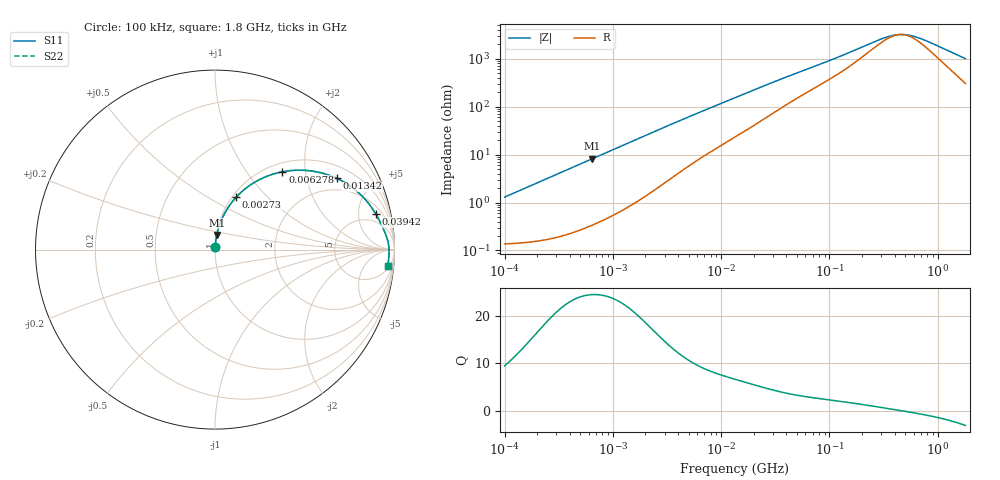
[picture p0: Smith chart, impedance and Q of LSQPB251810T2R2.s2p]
! LSQPB251810T2R2  S-PARAMETER MODEL  ( General Type )
! Model Generated by TAIYO YUDEN Corporation (http://www.ty-top.com)
! Version 2.0
! TAIYO YUDEN Control No. 100810NG22EB-FKC
! Copyright(c) 2009 TAIYO YUDEN CO.,LTD. All Rights Reserved.
! Product Description (link to TY-COMPAS)
! https://ds.yuden.co.jp/TYCOMPAS/or/detail?pn=LSQPB251810T2R2M&u=M
! Products Name : Inductors
! Characteristics :
!  Inductance : 2.2 uH , SRF(min) : 80 MHz , DC Resistance(max) : 0.169 Ohm
!  Rated Current : Saturation :850 mA , Temp Rise : 950 mA (40 degC)
!  Case Size : 2.5 x 1.8 / 0.098 x 0.071 [mm/inch] , Thickness : 1.0 / 0.04 [mm/inch]
!  (Conditions: Temperature = 25 degC , DC Bias Current/Voltage = 0A / 0V)
! External Node Assignments :
!  1  o---GGG---o  2
! GND o---------o GND
! Frequency Range : 0.1MHz  -  1800MHz  [ 402 STEP ]
# MHz S RI R 50
! Freq[MHz].  S11 Real  S11 Imag  S21 Real  S21 Imag  S12 Real  S12 Imag  S22 Real  S22 Imag
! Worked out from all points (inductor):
!   401 points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, 100 kHz to 1.8 GHz, reference 50 ohm
!   read as one part in series: L = 2.05 uH near 105 kHz
!   highest Q = 24.4 at 643.4 kHz (marker M1), where L = 2.03 uH
!   self-resonance near 452.5 MHz
!   S11 on the Smith chart (normalised r, x): 100 kHz: 1.00, +0.03; 2.73 MHz: 1.04, +0.68; 6.278 MHz: 1.16, +1.50; 13.42 MHz: 1.46, +3.03; 39.42 MHz: 3.14, +7.89; 1.8 GHz: 7, -19
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0.1  0.00153 0.0128  0.9985 -0.0128  0.9985 -0.0128  0.00153 0.0128
0.253659  0.00276 0.0324  0.9972 -0.0324  0.9972 -0.0324  0.00276 0.0324
0.516129  0.00703 0.0653  0.993 -0.0653  0.993 -0.0653  0.00703 0.0653
0.643431  0.00995 0.0809  0.99 -0.0809  0.99 -0.0809  0.00995 0.0809
1.479789  0.0414 0.177  0.9586 -0.177  0.9586 -0.177  0.0414 0.177
2.66389  0.114 0.2876  0.886 -0.2876  0.886 -0.2876  0.114 0.2876
2.729949  0.1187 0.2927  0.8813 -0.2927  0.8813 -0.2927  0.1187 0.2927
4.039851  0.2168 0.3727  0.7832 -0.3727  0.7832 -0.3727  0.2168 0.3727
6.278453  0.376 0.4337  0.624 -0.4337  0.624 -0.4337  0.376 0.4337
9.066201  0.5277 0.4392  0.4723 -0.4392  0.4723 -0.4392  0.5277 0.4392
13.41641  0.677 0.3978  0.323 -0.3978  0.323 -0.3978  0.677 0.3978
22.44079  0.8165 0.3013  0.1835 -0.3013  0.1835 -0.3013  0.8165 0.3013
39.41996  0.8957 0.1987  0.1043 -0.1987  0.1043 -0.1987  0.8957 0.1987
69.24595  0.9336 0.1258  0.0664 -0.1258  0.0664 -0.1258  0.9336 0.1258
144.3909  0.9586 0.0629  0.0414 -0.0629  0.0414 -0.0629  0.9586 0.0629
272.9811  0.9673 0.0248  0.0327 -0.0248  0.0327 -0.0248  0.9673 0.0248
357.3983  0.9689 0.0113  0.0311 -0.0113  0.0311 -0.0113  0.9689 0.0113
413.9822  0.9694 0.00424  0.0306 -0.00424  0.0306 -0.00424  0.9694 0.00424
467.921  0.9696 -0.00161  0.0304 0.00161  0.0304 0.00161  0.9696 -0.00161
612.6219  0.9698 -0.0148  0.0302 0.0148  0.0302 0.0148  0.9698 -0.0148
802.0705  0.9694 -0.029  0.0306 0.029  0.0306 0.029  0.9694 -0.029
1800  0.9623 -0.089  0.0377 0.089  0.0377 0.089  0.9623 -0.089
